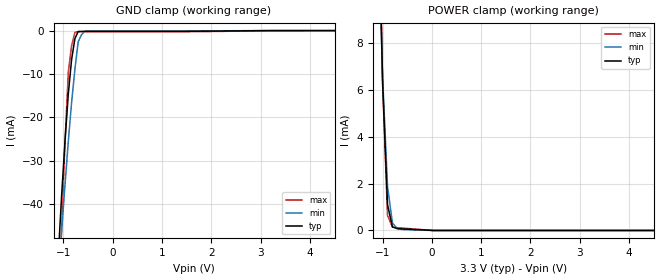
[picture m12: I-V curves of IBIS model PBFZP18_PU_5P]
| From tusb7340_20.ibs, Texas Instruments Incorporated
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|   Model Cell PBFZP18_PU_5P
|IC33SHYPBFZP18_PU_3P3
[Model]   PBFZP18_PU_5P
Model_type   Input
Polarity   Non-Inverting
Vinl =  0.8V
Vinh =  2V
C_comp   0.3896289p   0.3157674p   0.4571453p
[Model Spec]
Vinl   0.8V   0.8V   0.8V
Vinh   2V   2V   2V
[Temperature Range]   25   125   -40
[Voltage Range]   3.3   3.135   3.465
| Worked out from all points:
|   GND clamp passes 1 mA (typ) near -0.73 V on its own axis
|   POWER clamp passes 1 mA (typ) near -0.89 V on its own axis
[POWER_clamp]
|   voltage   I(typ)   I(min)   I(max)
-3.3V     301.3mA    233.2mA    387.8mA
-1.033V   9.499mA    8.962mA    10.24mA
-1V       6.393mA    6.577mA    6.309mA
-900mV    1.111mA    1.888mA    644.6uA
-800mV    151.7uA    320.3uA    146.8uA
-700mV    81.41uA    75.52uA    119.3uA
0V        0A         0A         0A
6.6V      0A         0A         0A
[GND_clamp]
|   voltage   I(typ)   I(min)   I(max)
-3.3V     -758.5mA   -699.4mA   -1.009A
-1.1V     -51.2mA    -56.69mA   -67.11mA
-1.033V   -37.59mA   -45.84mA   -44.88mA
-966.7mV  -25.38mA   -35.45mA   -25.69mA
-900mV    -14.56mA   -25.5mA    -9.536mA
-833.3mV  -6.657mA   -16.57mA   -3.497mA
-766.7mV  -1.875mA   -8.927mA   -410.2uA
-700mV    -213.4uA   -2.582mA   -275.9uA
-633.3mV  -187.2uA   -993.5uA   -274.9uA
-566.7mV  -174uA     -165.1uA   -274.3uA
6.6V      0A         0A         0A
